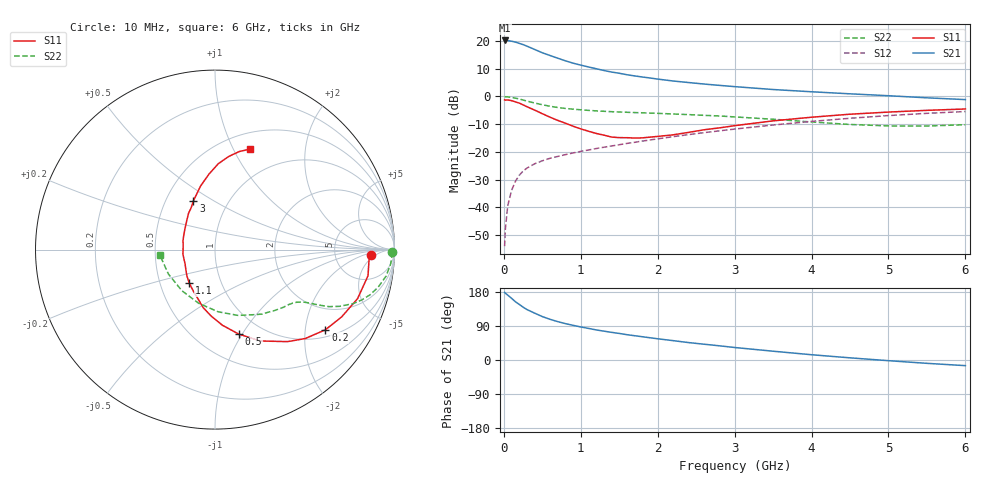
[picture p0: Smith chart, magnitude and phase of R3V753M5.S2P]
! SIEMENS Small Signal Semiconductors
! BFR181
! Si NPN RF Bipolar Junction Transistor in SOT23
! VCE = 0.75 V  IC = 3.5 mA
! Common Emitter S-Parameters:  May  1996
# GHz  S  MA  R  50
!  f  S11  S21  S12  S22
! GHz  MAG  ANG  MAG  ANG  MAG  ANG  MAG  ANG
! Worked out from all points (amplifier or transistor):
!   36 points, 10 MHz to 6 GHz, reference 50 ohm
!   highest |S21| = 20.2 dB at 10 MHz (marker M1)
!   |S21| within 3 dB of that: start of sweep to 380 MHz
!   unconditionally stable (mu >= 1): 1.106 GHz to 3.485 GHz
!   at 250 MHz: K = 0.36, MSG = 22.8 dB, |S12| = -26.9 dB
!   at 1.4 GHz: K = 1.08, MAG = 11.6 dB, |S12| = -17.9 dB
!   at 6 GHz: K = 0.91, MSG = 2.1 dB, |S12| = -5.4 dB
!   S11 on the Smith chart (normalised r, x): 10 MHz: 13, -3; 200 MHz: 1.21, -2.57; 500 MHz: 0.78, -0.97; 1.1 GHz: 0.70, -0.28; 3 GHz: 0.69, +0.41; 6 GHz: 0.67, +1.17
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0.01  0.8683 -2.1  10.23 178.4  0.002 89.8  0.9887 -0.9
0.02  0.8601 -3.8  10.2 176.3  0.0041 90.0  0.9868 -1.9
0.05  0.8649 -9.7  10.15 171.3  0.0106 82.9  0.9821 -4.6
0.1  0.8399 -19.0  9.929 162.9  0.0203 80.2  0.9646 -8.8
0.15  0.799 -28.0  9.557 153.8  0.0294 74.4  0.9334 -12.9
0.2  0.7601 -36.0  9.077 146.8  0.0379 70.9  0.9008 -16.2
0.25  0.7064 -44.5  8.616 139.5  0.0451 67.2  0.8636 -19.0
0.3  0.6534 -51.7  8.078 133.2  0.0511 64.5  0.8257 -21.4
0.4  0.5684 -63.6  7.044 123.7  0.0611 60.4  0.7622 -24.5
0.5  0.4891 -74.3  6.134 114.6  0.0692 58.5  0.7099 -26.6
0.6  0.4228 -84.5  5.477 107.4  0.0768 57.1  0.666 -27.8
0.7  0.3708 -93.3  4.901 101.3  0.0829 56.5  0.633 -28.7
0.8  0.33 -101.5  4.393 96.0  0.0894 56.0  0.6086 -29.4
1.1  0.2362 -127.3  3.403 83.4  0.1083 56.5  0.5613 -31.4
1.3  0.2008 -143.3  2.94 76.2  0.1216 57.1  0.5403 -32.9
1.6  0.1807 -171.7  2.465 66.8  0.1425 57.5  0.5188 -35.7
2.2  0.2032 145.6  1.901 51.1  0.1884 56.8  0.4835 -43.5
3  0.2975 113.8  1.504 33.0  0.2582 52.7  0.4279 -57.8
3.5  0.3631 102.8  1.334 23.2  0.3059 48.7  0.3885 -70.7
4.5  0.4788 87.8  1.116 5.7  0.4044 38.1  0.3127 -106.9
5.5  0.5622 76.2  0.945 -8.8  0.4964 25.2  0.2931 -152.5
6  0.5944 70.6  0.878 -14.9  0.5355 18.2  0.3094 -174.6
